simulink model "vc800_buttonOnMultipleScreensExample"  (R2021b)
settings: Solver=FixedStepDiscrete  StartTime=0.0  StopTime=10.0  FixedStep=0.01  RelTol=1e-3  EnableMultiTasking=on
PreLoadFcn:
  | try, model_open; catch, disp('Error occurred while executing model pre-load callback: model_open.m'); disp('Please assure that the MATLAB working directory is set to the model directory before opening.'); end
InitFcn:
  | try, model_open; catch, end
model workspace (MAT data in the model file):
  IOScreen_Label_XCoord = 1
  IOScreen_Row1_YCoord = 1
  IOScreen_Row2_YCoord = 12
  IOScreen_Value_XCoord = 110
  MainScreen_Row1_YCoord = 7
  MainScreen_Row2_YCoord = 23
  MainScreen_Symbols_XCoord = 1
  MainScreen_Units_XCoord = 69
  MainScreen_Value_XCoord = 64
undefined symbols (not defined in the file or in its folder): case, curr_screen, default, DISP, filtering, gesture, hex2dec, Mode, No, raptor_get_buildNum, raptor_get_safe_string, raptor_hwexp, raptor_xcp_function, Screens, VC800, Voltage
libraries: Raptor_display_lib x190, Raptor_lib x97, simulink_extras x11, Raptor_Datalogging_lib x10, simulink x2
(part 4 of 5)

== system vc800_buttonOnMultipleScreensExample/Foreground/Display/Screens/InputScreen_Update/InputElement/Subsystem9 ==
  y_start_offset : Inport
  x : Inport  Port=2
  In3 : Inport  Port=3
  in_value : Inport  Port=4
  Add22 : Sum
  Constant26 : Constant  Value=40  OutDataTypeStr=int32
  display_draw_text13 : Raptor_display_lib/Drawing Functions/display_draw_text  textPort=off  textVal=in_nam  colorPort=off  col=FFFF  opacity=100  font=Future  fontFile=''  heightPort=off  height=20  hAlign=Right  vAlign=Center  spacing=0  layer=Background  pnPort=off
  display_draw_text14 : Raptor_display_lib/Drawing Functions/display_draw_text  textPort=on  textVal='Input1'  colorPort=off  col=FFFF  opacity=100  font=Future  fontFile=''  heightPort=off  height=20  hAlign=Left  vAlign=Center  spacing=0  layer=Background  pnPort=off
  raptor_string : Raptor_lib/Strings/raptor_string  stringName=''  string=''  dynamicSize=Fixed Size  strSize=10  storage=Volatile (RAM)  calVisible=off  calAccess=4  strFunction=raptor_xcp_function(gcb)
  raptor_string_printf : Raptor_lib/Strings/raptor_string_printf  formatString='%u'
  y_end_offset : Outport  VectorParamsAs1DForOutWhenUnconnected=off
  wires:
  raptor_string/1 -> raptor_string_printf/1
  Add22/1 -> display_draw_text13/2, y_end_offset/1, display_draw_text14/2
  In3/1 -> display_draw_text14/1
  raptor_string_printf/1 -> display_draw_text14/3
  y_start_offset/1 -> Add22/1
  Constant26/1 -> Add22/2
  in_value/1 -> raptor_string_printf/2
  x/1 -> display_draw_text13/1

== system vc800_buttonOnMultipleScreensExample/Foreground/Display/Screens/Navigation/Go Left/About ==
  Action Port : ActionPort  ActionPortLabel=case [ 5 ]:
  display_goto_screen : Raptor_display_lib/Screen Functions/display_goto_screen  screenPort=off  ScreenName='MainScreen'

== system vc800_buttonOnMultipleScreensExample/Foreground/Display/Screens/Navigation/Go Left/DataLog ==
  Action Port : ActionPort  ActionPortLabel=case [ 4 ]:
  display_goto_screen : Raptor_display_lib/Screen Functions/display_goto_screen  screenPort=off  ScreenName='AboutScreen'

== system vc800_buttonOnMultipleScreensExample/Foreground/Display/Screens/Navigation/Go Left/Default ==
  Action Port : ActionPort  ActionPortLabel=default:
  display_goto_screen : Raptor_display_lib/Screen Functions/display_goto_screen  screenPort=off  ScreenName='MainScreen'

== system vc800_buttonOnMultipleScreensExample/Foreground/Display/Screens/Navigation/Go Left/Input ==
  Action Port : ActionPort  ActionPortLabel=case [ 2 ]:
  display_goto_screen : Raptor_display_lib/Screen Functions/display_goto_screen  screenPort=off  ScreenName='OutputScreen'

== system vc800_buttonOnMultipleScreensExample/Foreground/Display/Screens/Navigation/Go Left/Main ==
  Action Port : ActionPort  ActionPortLabel=case [ 1 ]:
  display_goto_screen : Raptor_display_lib/Screen Functions/display_goto_screen  screenPort=off  ScreenName='InputScreen'

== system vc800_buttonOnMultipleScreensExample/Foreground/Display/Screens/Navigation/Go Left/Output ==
  Action Port : ActionPort  ActionPortLabel=case [ 3 ]:
  display_goto_screen : Raptor_display_lib/Screen Functions/display_goto_screen  screenPort=off  ScreenName='DataLogScreen'

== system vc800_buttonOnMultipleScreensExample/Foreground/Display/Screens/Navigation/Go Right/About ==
  Action Port : ActionPort  ActionPortLabel=case [ 5 ]:
  display_goto_screen : Raptor_display_lib/Screen Functions/display_goto_screen  screenPort=off  ScreenName='DataLogScreen'

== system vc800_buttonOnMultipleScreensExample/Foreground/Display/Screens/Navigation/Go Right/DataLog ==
  Action Port : ActionPort  ActionPortLabel=case [ 4 ]:
  display_goto_screen : Raptor_display_lib/Screen Functions/display_goto_screen  screenPort=off  ScreenName='OutputScreen'

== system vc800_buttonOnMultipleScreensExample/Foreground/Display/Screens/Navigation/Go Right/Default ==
  Action Port : ActionPort  ActionPortLabel=default:
  display_goto_screen : Raptor_display_lib/Screen Functions/display_goto_screen  screenPort=off  ScreenName='MainScreen'

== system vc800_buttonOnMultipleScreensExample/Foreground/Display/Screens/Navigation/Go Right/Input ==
  Action Port : ActionPort  ActionPortLabel=case [ 2 ]:
  display_goto_screen : Raptor_display_lib/Screen Functions/display_goto_screen  screenPort=off  ScreenName='MainScreen'

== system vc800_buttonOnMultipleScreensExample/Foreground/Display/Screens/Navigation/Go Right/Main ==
  Action Port : ActionPort  ActionPortLabel=case [ 1 ]:
  display_goto_screen : Raptor_display_lib/Screen Functions/display_goto_screen  screenPort=off  ScreenName='AboutScreen'

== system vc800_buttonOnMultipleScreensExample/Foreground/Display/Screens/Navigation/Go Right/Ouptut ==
  Action Port : ActionPort  ActionPortLabel=case [ 3 ]:
  display_goto_screen : Raptor_display_lib/Screen Functions/display_goto_screen  screenPort=off  ScreenName='InputScreen'

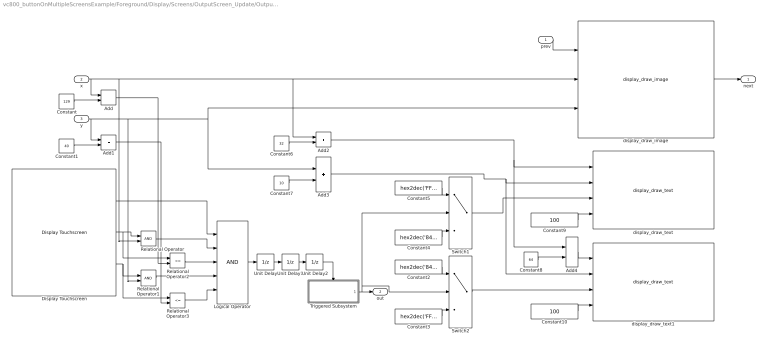
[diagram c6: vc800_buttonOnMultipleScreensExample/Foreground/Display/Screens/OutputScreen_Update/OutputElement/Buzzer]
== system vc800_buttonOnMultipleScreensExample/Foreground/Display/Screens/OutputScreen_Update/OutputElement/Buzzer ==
  prev : Inport
  x : Inport  Port=2
  y : Inport  Port=3
  Add{,1..4} (5 alike) : Sum
  Constant : Constant  Value=129
  Constant1 : Constant  Value=40
  Constant10 : Constant  Value=100  OutDataTypeStr=uint32
  Constant2 : Constant  Value=hex2dec('8410')  OutDataTypeStr=uint16
  Constant3 : Constant  Value=hex2dec('FFFF')  OutDataTypeStr=uint16
  Constant4 : Constant  Value=hex2dec('8410')  OutDataTypeStr=uint16
  Constant5 : Constant  Value=hex2dec('FFFF')  OutDataTypeStr=uint16
  Constant6 : Constant  Value=32  OutDataTypeStr=int32
  Constant7 : Constant  Value=10  OutDataTypeStr=int32
  Constant8 : Constant  Value=64  OutDataTypeStr=int32
  Constant9 : Constant  Value=100  OutDataTypeStr=uint32
  Display Touchscreen : Raptor_display_lib/Touchscreen/Display Touchscreen
  Logical Operator : Logic  Inputs=5  IconShape=distinctive  AllPortsSameDT=off  OutDataTypeStr=boolean
  Relational Operator : RelationalOperator  OutDataTypeStr=boolean
  Relational Operator1 : RelationalOperator  OutDataTypeStr=boolean
  Relational Operator2 : RelationalOperator  Operator=<=  OutDataTypeStr=boolean
  Relational Operator3 : RelationalOperator  Operator=<=  OutDataTypeStr=boolean
  Switch1 : Switch  Criteria=u2 ~= 0
  Switch2 : Switch  Criteria=u2 ~= 0
  Triggered Subsystem : Subsystem  TreatAsAtomicUnit=on
  Unit Delay : UnitDelay  SampleTime=-1  HasFrameUpgradeWarning=on
  Unit Delay1 : UnitDelay  InitialCondition=1  SampleTime=-1  HasFrameUpgradeWarning=on
  Unit Delay2 : UnitDelay  SampleTime=-1  HasFrameUpgradeWarning=on
  display_draw_image : Raptor_display_lib/Drawing Functions/display_draw_image  imagePort=off  imageFile=toggle_frame.png  opacityPort=off  opacity=100  drawMode=Draw Entire Image  alpha=Draw as Transparent  layer=Background  drawModeXY=Top Left  pnPort=on
  display_draw_text : Raptor_display_lib/Drawing Functions/display_draw_text  textPort=off  textVal='On'  colorPort=on  col=8410  opacity=100  font=Future  fontFile=''  heightPort=off  height=20  hAlign=Center  vAlign=Top  spacing=0  layer=Background  pnPort=off
  display_draw_text1 : Raptor_display_lib/Drawing Functions/display_draw_text  textPort=off  textVal='Off'  colorPort=on  col=FFFF  opacity=100  font=Future  fontFile=''  heightPort=off  height=20  hAlign=Center  vAlign=Top  spacing=0  layer=Background  pnPort=off
  next : Outport  VectorParamsAs1DForOutWhenUnconnected=off
  out : Outport  Port=2  VectorParamsAs1DForOutWhenUnconnected=off
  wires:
  x/1 -> Add/1, Relational Operator/2, Add2/1, display_draw_image/2
  Display Touchscreen/2 -> Relational Operator/1, Relational Operator2/1
  Display Touchscreen/3 -> Relational Operator1/1, Relational Operator3/1
  y/1 -> Add1/1, Relational Operator1/2, Add3/1, display_draw_image/3
  Constant/1 -> Add/2
  Constant1/1 -> Add1/2
  Add/1 -> Relational Operator2/2
  Add1/1 -> Relational Operator3/2
  Relational Operator3/1 -> Logical Operator/5
  Relational Operator1/1 -> Logical Operator/4
  Relational Operator2/1 -> Logical Operator/3
  Relational Operator/1 -> Logical Operator/2
  Display Touchscreen/1 -> Logical Operator/1
  Unit Delay1/1 -> Unit Delay2/1
  Unit Delay/1 -> Unit Delay1/1
  Logical Operator/1 -> Unit Delay/1
  Unit Delay2/1 -> Triggered Subsystem/Trigger
  prev/1 -> display_draw_image/1
  display_draw_image/1 -> next/1
  Triggered Subsystem/1(Out1) -> Switch1/2, Switch2/2, out/1
  Switch1/1 -> display_draw_text/3
  Switch2/1 -> display_draw_text1/3
  Constant2/1 -> Switch2/1
  Constant4/1 -> Switch1/3
  Constant3/1 -> Switch2/3
  Constant5/1 -> Switch1/1
  Constant6/1 -> Add2/2
  Add2/1 -> Add4/1, display_draw_text/1
  Constant7/1 -> Add3/2
  Add3/1 -> display_draw_text/2, display_draw_text1/2
  Constant8/1 -> Add4/2
  Add4/1 -> display_draw_text1/1
  Constant9/1 -> display_draw_text/4
  Constant10/1 -> display_draw_text1/4

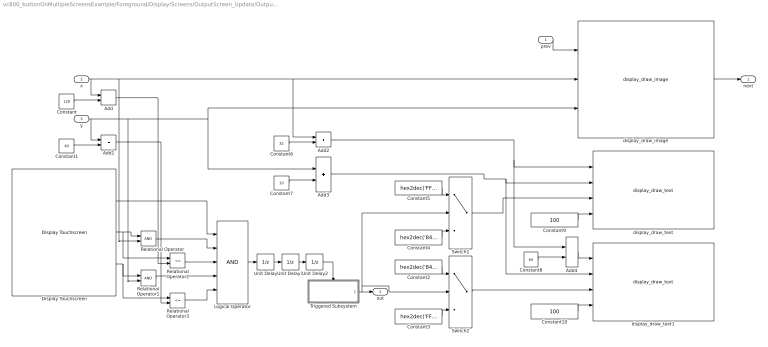
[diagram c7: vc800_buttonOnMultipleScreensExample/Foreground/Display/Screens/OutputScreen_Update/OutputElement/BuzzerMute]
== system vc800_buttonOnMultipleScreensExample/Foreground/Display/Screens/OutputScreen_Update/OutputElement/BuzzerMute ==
  prev : Inport
  x : Inport  Port=2
  y : Inport  Port=3
  Add{,1..4} (5 alike) : Sum
  Constant : Constant  Value=129
  Constant1 : Constant  Value=40
  Constant10 : Constant  Value=100  OutDataTypeStr=uint32
  Constant2 : Constant  Value=hex2dec('8410')  OutDataTypeStr=uint16
  Constant3 : Constant  Value=hex2dec('FFFF')  OutDataTypeStr=uint16
  Constant4 : Constant  Value=hex2dec('8410')  OutDataTypeStr=uint16
  Constant5 : Constant  Value=hex2dec('FFFF')  OutDataTypeStr=uint16
  Constant6 : Constant  Value=32  OutDataTypeStr=int32
  Constant7 : Constant  Value=10  OutDataTypeStr=int32
  Constant8 : Constant  Value=64  OutDataTypeStr=int32
  Constant9 : Constant  Value=100  OutDataTypeStr=uint32
  Display Touchscreen : Raptor_display_lib/Touchscreen/Display Touchscreen
  Logical Operator : Logic  Inputs=5  IconShape=distinctive  AllPortsSameDT=off  OutDataTypeStr=boolean
  Relational Operator : RelationalOperator  OutDataTypeStr=boolean
  Relational Operator1 : RelationalOperator  OutDataTypeStr=boolean
  Relational Operator2 : RelationalOperator  Operator=<=  OutDataTypeStr=boolean
  Relational Operator3 : RelationalOperator  Operator=<=  OutDataTypeStr=boolean
  Switch1 : Switch  Criteria=u2 ~= 0
  Switch2 : Switch  Criteria=u2 ~= 0
  Triggered Subsystem : Subsystem  TreatAsAtomicUnit=on
  Unit Delay : UnitDelay  SampleTime=-1  HasFrameUpgradeWarning=on
  Unit Delay1 : UnitDelay  InitialCondition=1  SampleTime=-1  HasFrameUpgradeWarning=on
  Unit Delay2 : UnitDelay  SampleTime=-1  HasFrameUpgradeWarning=on
  display_draw_image : Raptor_display_lib/Drawing Functions/display_draw_image  imagePort=off  imageFile=toggle_frame.png  opacityPort=off  opacity=100  drawMode=Draw Entire Image  alpha=Draw as Transparent  layer=Background  drawModeXY=Top Left  pnPort=on
  display_draw_text : Raptor_display_lib/Drawing Functions/display_draw_text  textPort=off  textVal='On'  colorPort=on  col=8410  opacity=100  font=Future  fontFile=''  heightPort=off  height=20  hAlign=Center  vAlign=Top  spacing=0  layer=Background  pnPort=off
  display_draw_text1 : Raptor_display_lib/Drawing Functions/display_draw_text  textPort=off  textVal='Off'  colorPort=on  col=FFFF  opacity=100  font=Future  fontFile=''  heightPort=off  height=20  hAlign=Center  vAlign=Top  spacing=0  layer=Background  pnPort=off
  next : Outport  VectorParamsAs1DForOutWhenUnconnected=off
  out : Outport  Port=2  VectorParamsAs1DForOutWhenUnconnected=off
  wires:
  Constant10/1 -> display_draw_text1/4
  Constant9/1 -> display_draw_text/4
  Add4/1 -> display_draw_text1/1
  Constant8/1 -> Add4/2
  Add3/1 -> display_draw_text1/2, display_draw_text/2
  Constant7/1 -> Add3/2
  Add2/1 -> display_draw_text/1, Add4/1
  Constant6/1 -> Add2/2
  Constant5/1 -> Switch1/1
  Constant3/1 -> Switch2/3
  Constant4/1 -> Switch1/3
  Constant2/1 -> Switch2/1
  Switch2/1 -> display_draw_text1/3
  Switch1/1 -> display_draw_text/3
  Triggered Subsystem/1(Out1) -> out/1, Switch2/2, Switch1/2
  display_draw_image/1 -> next/1
  prev/1 -> display_draw_image/1
  Unit Delay2/1 -> Triggered Subsystem/Trigger
  Logical Operator/1 -> Unit Delay/1
  Unit Delay/1 -> Unit Delay1/1
  Unit Delay1/1 -> Unit Delay2/1
  Display Touchscreen/1 -> Logical Operator/1
  Relational Operator/1 -> Logical Operator/2
  Relational Operator2/1 -> Logical Operator/3
  Relational Operator1/1 -> Logical Operator/4
  Relational Operator3/1 -> Logical Operator/5
  Add1/1 -> Relational Operator3/2
  Add/1 -> Relational Operator2/2
  Constant1/1 -> Add1/2
  Constant/1 -> Add/2
  y/1 -> display_draw_image/3, Add3/1, Relational Operator1/2, Add1/1
  Display Touchscreen/3 -> Relational Operator3/1, Relational Operator1/1
  Display Touchscreen/2 -> Relational Operator2/1, Relational Operator/1
  x/1 -> display_draw_image/2, Add2/1, Relational Operator/2, Add/1

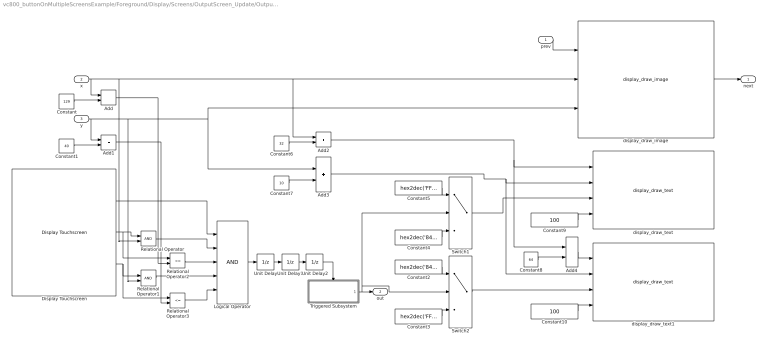
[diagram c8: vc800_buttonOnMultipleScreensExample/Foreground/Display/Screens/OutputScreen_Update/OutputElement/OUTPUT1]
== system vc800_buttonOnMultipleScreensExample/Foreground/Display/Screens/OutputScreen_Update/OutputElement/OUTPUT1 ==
  prev : Inport
  x : Inport  Port=2
  y : Inport  Port=3
  Add{,1..4} (5 alike) : Sum
  Constant : Constant  Value=129
  Constant1 : Constant  Value=40
  Constant10 : Constant  Value=100  OutDataTypeStr=uint32
  Constant2 : Constant  Value=hex2dec('8410')  OutDataTypeStr=uint16
  Constant3 : Constant  Value=hex2dec('FFFF')  OutDataTypeStr=uint16
  Constant4 : Constant  Value=hex2dec('8410')  OutDataTypeStr=uint16
  Constant5 : Constant  Value=hex2dec('FFFF')  OutDataTypeStr=uint16
  Constant6 : Constant  Value=32  OutDataTypeStr=int32
  Constant7 : Constant  Value=10  OutDataTypeStr=int32
  Constant8 : Constant  Value=64  OutDataTypeStr=int32
  Constant9 : Constant  Value=100  OutDataTypeStr=uint32
  Display Touchscreen : Raptor_display_lib/Touchscreen/Display Touchscreen
  Logical Operator : Logic  Inputs=5  IconShape=distinctive  AllPortsSameDT=off  OutDataTypeStr=boolean
  Relational Operator : RelationalOperator  OutDataTypeStr=boolean
  Relational Operator1 : RelationalOperator  OutDataTypeStr=boolean
  Relational Operator2 : RelationalOperator  Operator=<=  OutDataTypeStr=boolean
  Relational Operator3 : RelationalOperator  Operator=<=  OutDataTypeStr=boolean
  Switch1 : Switch  Criteria=u2 ~= 0
  Switch2 : Switch  Criteria=u2 ~= 0
  Triggered Subsystem : Subsystem  TreatAsAtomicUnit=on
  Unit Delay : UnitDelay  SampleTime=-1  HasFrameUpgradeWarning=on
  Unit Delay1 : UnitDelay  InitialCondition=1  SampleTime=-1  HasFrameUpgradeWarning=on
  Unit Delay2 : UnitDelay  SampleTime=-1  HasFrameUpgradeWarning=on
  display_draw_image : Raptor_display_lib/Drawing Functions/display_draw_image  imagePort=off  imageFile=toggle_frame.png  opacityPort=off  opacity=100  drawMode=Draw Entire Image  alpha=Draw as Transparent  layer=Background  drawModeXY=Top Left  pnPort=on
  display_draw_text : Raptor_display_lib/Drawing Functions/display_draw_text  textPort=off  textVal='On'  colorPort=on  col=8410  opacity=100  font=Future  fontFile=''  heightPort=off  height=20  hAlign=Center  vAlign=Top  spacing=0  layer=Background  pnPort=off
  display_draw_text1 : Raptor_display_lib/Drawing Functions/display_draw_text  textPort=off  textVal='Off'  colorPort=on  col=FFFF  opacity=100  font=Future  fontFile=''  heightPort=off  height=20  hAlign=Center  vAlign=Top  spacing=0  layer=Background  pnPort=off
  next : Outport  VectorParamsAs1DForOutWhenUnconnected=off
  out : Outport  Port=2  VectorParamsAs1DForOutWhenUnconnected=off
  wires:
  x/1 -> Add/1, Relational Operator/2, Add2/1, display_draw_image/2
  Display Touchscreen/2 -> Relational Operator/1, Relational Operator2/1
  Display Touchscreen/3 -> Relational Operator1/1, Relational Operator3/1
  y/1 -> Add1/1, Relational Operator1/2, Add3/1, display_draw_image/3
  Constant/1 -> Add/2
  Constant1/1 -> Add1/2
  Add/1 -> Relational Operator2/2
  Add1/1 -> Relational Operator3/2
  Relational Operator3/1 -> Logical Operator/5
  Relational Operator1/1 -> Logical Operator/4
  Relational Operator2/1 -> Logical Operator/3
  Relational Operator/1 -> Logical Operator/2
  Display Touchscreen/1 -> Logical Operator/1
  Unit Delay1/1 -> Unit Delay2/1
  Unit Delay/1 -> Unit Delay1/1
  Logical Operator/1 -> Unit Delay/1
  Unit Delay2/1 -> Triggered Subsystem/Trigger
  prev/1 -> display_draw_image/1
  display_draw_image/1 -> next/1
  Triggered Subsystem/1(Out1) -> Switch1/2, Switch2/2, out/1
  Switch1/1 -> display_draw_text/3
  Switch2/1 -> display_draw_text1/3
  Constant2/1 -> Switch2/1
  Constant4/1 -> Switch1/3
  Constant3/1 -> Switch2/3
  Constant5/1 -> Switch1/1
  Constant6/1 -> Add2/2
  Add2/1 -> Add4/1, display_draw_text/1
  Constant7/1 -> Add3/2
  Add3/1 -> display_draw_text/2, display_draw_text1/2
  Constant8/1 -> Add4/2
  Add4/1 -> display_draw_text1/1
  Constant9/1 -> display_draw_text/4
  Constant10/1 -> display_draw_text1/4

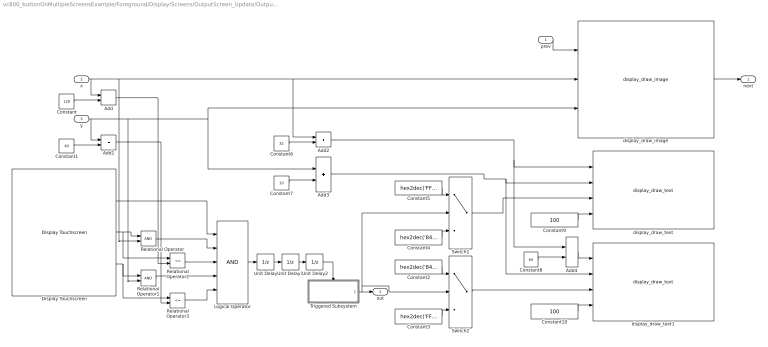
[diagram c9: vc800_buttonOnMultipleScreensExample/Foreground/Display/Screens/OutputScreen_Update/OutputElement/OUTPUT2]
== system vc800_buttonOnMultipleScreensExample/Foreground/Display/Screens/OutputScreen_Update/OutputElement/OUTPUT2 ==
  prev : Inport
  x : Inport  Port=2
  y : Inport  Port=3
  Add{,1..4} (5 alike) : Sum
  Constant : Constant  Value=129
  Constant1 : Constant  Value=40
  Constant10 : Constant  Value=100  OutDataTypeStr=uint32
  Constant2 : Constant  Value=hex2dec('8410')  OutDataTypeStr=uint16
  Constant3 : Constant  Value=hex2dec('FFFF')  OutDataTypeStr=uint16
  Constant4 : Constant  Value=hex2dec('8410')  OutDataTypeStr=uint16
  Constant5 : Constant  Value=hex2dec('FFFF')  OutDataTypeStr=uint16
  Constant6 : Constant  Value=32  OutDataTypeStr=int32
  Constant7 : Constant  Value=10  OutDataTypeStr=int32
  Constant8 : Constant  Value=64  OutDataTypeStr=int32
  Constant9 : Constant  Value=100  OutDataTypeStr=uint32
  Display Touchscreen : Raptor_display_lib/Touchscreen/Display Touchscreen
  Logical Operator : Logic  Inputs=5  IconShape=distinctive  AllPortsSameDT=off  OutDataTypeStr=boolean
  Relational Operator : RelationalOperator  OutDataTypeStr=boolean
  Relational Operator1 : RelationalOperator  OutDataTypeStr=boolean
  Relational Operator2 : RelationalOperator  Operator=<=  OutDataTypeStr=boolean
  Relational Operator3 : RelationalOperator  Operator=<=  OutDataTypeStr=boolean
  Switch1 : Switch  Criteria=u2 ~= 0
  Switch2 : Switch  Criteria=u2 ~= 0
  Triggered Subsystem : Subsystem  TreatAsAtomicUnit=on
  Unit Delay : UnitDelay  SampleTime=-1  HasFrameUpgradeWarning=on
  Unit Delay1 : UnitDelay  InitialCondition=1  SampleTime=-1  HasFrameUpgradeWarning=on
  Unit Delay2 : UnitDelay  SampleTime=-1  HasFrameUpgradeWarning=on
  display_draw_image : Raptor_display_lib/Drawing Functions/display_draw_image  imagePort=off  imageFile=toggle_frame.png  opacityPort=off  opacity=100  drawMode=Draw Entire Image  alpha=Draw as Transparent  layer=Background  drawModeXY=Top Left  pnPort=on
  display_draw_text : Raptor_display_lib/Drawing Functions/display_draw_text  textPort=off  textVal='On'  colorPort=on  col=8410  opacity=100  font=Future  fontFile=''  heightPort=off  height=20  hAlign=Center  vAlign=Top  spacing=0  layer=Background  pnPort=off
  display_draw_text1 : Raptor_display_lib/Drawing Functions/display_draw_text  textPort=off  textVal='Off'  colorPort=on  col=FFFF  opacity=100  font=Future  fontFile=''  heightPort=off  height=20  hAlign=Center  vAlign=Top  spacing=0  layer=Background  pnPort=off
  next : Outport  VectorParamsAs1DForOutWhenUnconnected=off
  out : Outport  Port=2  VectorParamsAs1DForOutWhenUnconnected=off
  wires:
  Constant10/1 -> display_draw_text1/4
  Constant9/1 -> display_draw_text/4
  Add4/1 -> display_draw_text1/1
  Constant8/1 -> Add4/2
  Add3/1 -> display_draw_text1/2, display_draw_text/2
  Constant7/1 -> Add3/2
  Add2/1 -> display_draw_text/1, Add4/1
  Constant6/1 -> Add2/2
  Constant5/1 -> Switch1/1
  Constant3/1 -> Switch2/3
  Constant4/1 -> Switch1/3
  Constant2/1 -> Switch2/1
  Switch2/1 -> display_draw_text1/3
  Switch1/1 -> display_draw_text/3
  Triggered Subsystem/1(Out1) -> out/1, Switch2/2, Switch1/2
  display_draw_image/1 -> next/1
  prev/1 -> display_draw_image/1
  Unit Delay2/1 -> Triggered Subsystem/Trigger
  Logical Operator/1 -> Unit Delay/1
  Unit Delay/1 -> Unit Delay1/1
  Unit Delay1/1 -> Unit Delay2/1
  Display Touchscreen/1 -> Logical Operator/1
  Relational Operator/1 -> Logical Operator/2
  Relational Operator2/1 -> Logical Operator/3
  Relational Operator1/1 -> Logical Operator/4
  Relational Operator3/1 -> Logical Operator/5
  Add1/1 -> Relational Operator3/2
  Add/1 -> Relational Operator2/2
  Constant1/1 -> Add1/2
  Constant/1 -> Add/2
  y/1 -> display_draw_image/3, Add3/1, Relational Operator1/2, Add1/1
  Display Touchscreen/3 -> Relational Operator3/1, Relational Operator1/1
  Display Touchscreen/2 -> Relational Operator2/1, Relational Operator/1
  x/1 -> display_draw_image/2, Add2/1, Relational Operator/2, Add/1

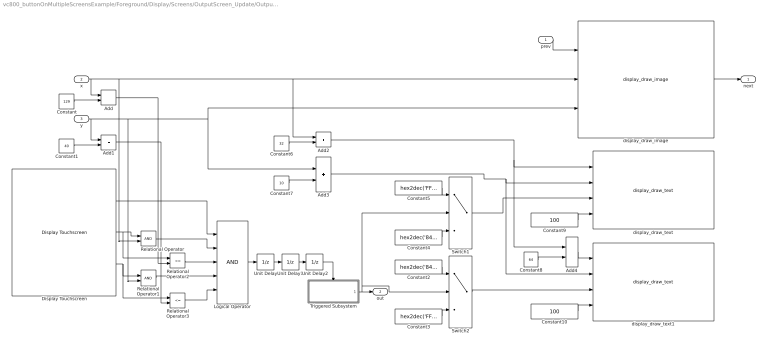
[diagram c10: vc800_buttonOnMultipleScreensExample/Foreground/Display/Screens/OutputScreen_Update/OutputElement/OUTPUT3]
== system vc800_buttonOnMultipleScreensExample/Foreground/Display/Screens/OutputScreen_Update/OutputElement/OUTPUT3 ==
  prev : Inport
  x : Inport  Port=2
  y : Inport  Port=3
  Add{,1..4} (5 alike) : Sum
  Constant : Constant  Value=129
  Constant1 : Constant  Value=40
  Constant10 : Constant  Value=100  OutDataTypeStr=uint32
  Constant2 : Constant  Value=hex2dec('8410')  OutDataTypeStr=uint16
  Constant3 : Constant  Value=hex2dec('FFFF')  OutDataTypeStr=uint16
  Constant4 : Constant  Value=hex2dec('8410')  OutDataTypeStr=uint16
  Constant5 : Constant  Value=hex2dec('FFFF')  OutDataTypeStr=uint16
  Constant6 : Constant  Value=32  OutDataTypeStr=int32
  Constant7 : Constant  Value=10  OutDataTypeStr=int32
  Constant8 : Constant  Value=64  OutDataTypeStr=int32
  Constant9 : Constant  Value=100  OutDataTypeStr=uint32
  Display Touchscreen : Raptor_display_lib/Touchscreen/Display Touchscreen
  Logical Operator : Logic  Inputs=5  IconShape=distinctive  AllPortsSameDT=off  OutDataTypeStr=boolean
  Relational Operator : RelationalOperator  OutDataTypeStr=boolean
  Relational Operator1 : RelationalOperator  OutDataTypeStr=boolean
  Relational Operator2 : RelationalOperator  Operator=<=  OutDataTypeStr=boolean
  Relational Operator3 : RelationalOperator  Operator=<=  OutDataTypeStr=boolean
  Switch1 : Switch  Criteria=u2 ~= 0
  Switch2 : Switch  Criteria=u2 ~= 0
  Triggered Subsystem : Subsystem  TreatAsAtomicUnit=on
  Unit Delay : UnitDelay  SampleTime=-1  HasFrameUpgradeWarning=on
  Unit Delay1 : UnitDelay  InitialCondition=1  SampleTime=-1  HasFrameUpgradeWarning=on
  Unit Delay2 : UnitDelay  SampleTime=-1  HasFrameUpgradeWarning=on
  display_draw_image : Raptor_display_lib/Drawing Functions/display_draw_image  imagePort=off  imageFile=toggle_frame.png  opacityPort=off  opacity=100  drawMode=Draw Entire Image  alpha=Draw as Transparent  layer=Background  drawModeXY=Top Left  pnPort=on
  display_draw_text : Raptor_display_lib/Drawing Functions/display_draw_text  textPort=off  textVal='On'  colorPort=on  col=8410  opacity=100  font=Future  fontFile=''  heightPort=off  height=20  hAlign=Center  vAlign=Top  spacing=0  layer=Background  pnPort=off
  display_draw_text1 : Raptor_display_lib/Drawing Functions/display_draw_text  textPort=off  textVal='Off'  colorPort=on  col=FFFF  opacity=100  font=Future  fontFile=''  heightPort=off  height=20  hAlign=Center  vAlign=Top  spacing=0  layer=Background  pnPort=off
  next : Outport  VectorParamsAs1DForOutWhenUnconnected=off
  out : Outport  Port=2  VectorParamsAs1DForOutWhenUnconnected=off
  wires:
  x/1 -> Add/1, Relational Operator/2, Add2/1, display_draw_image/2
  Display Touchscreen/2 -> Relational Operator/1, Relational Operator2/1
  Display Touchscreen/3 -> Relational Operator1/1, Relational Operator3/1
  y/1 -> Add1/1, Relational Operator1/2, Add3/1, display_draw_image/3
  Constant/1 -> Add/2
  Constant1/1 -> Add1/2
  Add/1 -> Relational Operator2/2
  Add1/1 -> Relational Operator3/2
  Relational Operator3/1 -> Logical Operator/5
  Relational Operator1/1 -> Logical Operator/4
  Relational Operator2/1 -> Logical Operator/3
  Relational Operator/1 -> Logical Operator/2
  Display Touchscreen/1 -> Logical Operator/1
  Unit Delay1/1 -> Unit Delay2/1
  Unit Delay/1 -> Unit Delay1/1
  Logical Operator/1 -> Unit Delay/1
  Unit Delay2/1 -> Triggered Subsystem/Trigger
  prev/1 -> display_draw_image/1
  display_draw_image/1 -> next/1
  Triggered Subsystem/1(Out1) -> Switch1/2, Switch2/2, out/1
  Switch1/1 -> display_draw_text/3
  Switch2/1 -> display_draw_text1/3
  Constant2/1 -> Switch2/1
  Constant4/1 -> Switch1/3
  Constant3/1 -> Switch2/3
  Constant5/1 -> Switch1/1
  Constant6/1 -> Add2/2
  Add2/1 -> Add4/1, display_draw_text/1
  Constant7/1 -> Add3/2
  Add3/1 -> display_draw_text/2, display_draw_text1/2
  Constant8/1 -> Add4/2
  Add4/1 -> display_draw_text1/1
  Constant9/1 -> display_draw_text/4
  Constant10/1 -> display_draw_text1/4

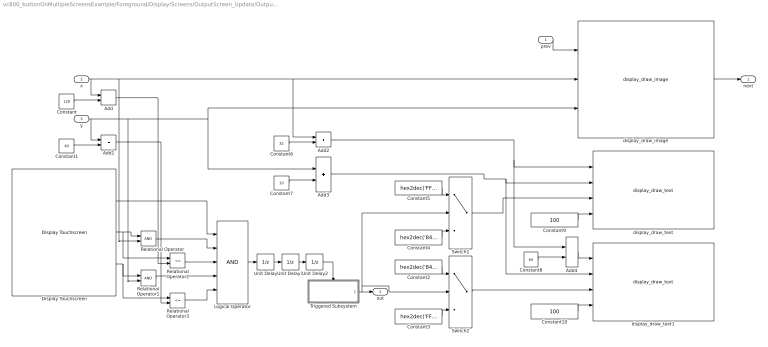
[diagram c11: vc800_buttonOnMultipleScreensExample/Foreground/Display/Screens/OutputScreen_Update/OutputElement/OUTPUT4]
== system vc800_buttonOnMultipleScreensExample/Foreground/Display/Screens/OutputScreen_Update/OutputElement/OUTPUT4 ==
  prev : Inport
  x : Inport  Port=2
  y : Inport  Port=3
  Add{,1..4} (5 alike) : Sum
  Constant : Constant  Value=129
  Constant1 : Constant  Value=40
  Constant10 : Constant  Value=100  OutDataTypeStr=uint32
  Constant2 : Constant  Value=hex2dec('8410')  OutDataTypeStr=uint16
  Constant3 : Constant  Value=hex2dec('FFFF')  OutDataTypeStr=uint16
  Constant4 : Constant  Value=hex2dec('8410')  OutDataTypeStr=uint16
  Constant5 : Constant  Value=hex2dec('FFFF')  OutDataTypeStr=uint16
  Constant6 : Constant  Value=32  OutDataTypeStr=int32
  Constant7 : Constant  Value=10  OutDataTypeStr=int32
  Constant8 : Constant  Value=64  OutDataTypeStr=int32
  Constant9 : Constant  Value=100  OutDataTypeStr=uint32
  Display Touchscreen : Raptor_display_lib/Touchscreen/Display Touchscreen
  Logical Operator : Logic  Inputs=5  IconShape=distinctive  AllPortsSameDT=off  OutDataTypeStr=boolean
  Relational Operator : RelationalOperator  OutDataTypeStr=boolean
  Relational Operator1 : RelationalOperator  OutDataTypeStr=boolean
  Relational Operator2 : RelationalOperator  Operator=<=  OutDataTypeStr=boolean
  Relational Operator3 : RelationalOperator  Operator=<=  OutDataTypeStr=boolean
  Switch1 : Switch  Criteria=u2 ~= 0
  Switch2 : Switch  Criteria=u2 ~= 0
  Triggered Subsystem : Subsystem  TreatAsAtomicUnit=on
  Unit Delay : UnitDelay  SampleTime=-1  HasFrameUpgradeWarning=on
  Unit Delay1 : UnitDelay  InitialCondition=1  SampleTime=-1  HasFrameUpgradeWarning=on
  Unit Delay2 : UnitDelay  SampleTime=-1  HasFrameUpgradeWarning=on
  display_draw_image : Raptor_display_lib/Drawing Functions/display_draw_image  imagePort=off  imageFile=toggle_frame.png  opacityPort=off  opacity=100  drawMode=Draw Entire Image  alpha=Draw as Transparent  layer=Background  drawModeXY=Top Left  pnPort=on
  display_draw_text : Raptor_display_lib/Drawing Functions/display_draw_text  textPort=off  textVal='On'  colorPort=on  col=8410  opacity=100  font=Future  fontFile=''  heightPort=off  height=20  hAlign=Center  vAlign=Top  spacing=0  layer=Background  pnPort=off
  display_draw_text1 : Raptor_display_lib/Drawing Functions/display_draw_text  textPort=off  textVal='Off'  colorPort=on  col=FFFF  opacity=100  font=Future  fontFile=''  heightPort=off  height=20  hAlign=Center  vAlign=Top  spacing=0  layer=Background  pnPort=off
  next : Outport  VectorParamsAs1DForOutWhenUnconnected=off
  out : Outport  Port=2  VectorParamsAs1DForOutWhenUnconnected=off
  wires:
  Constant10/1 -> display_draw_text1/4
  Constant9/1 -> display_draw_text/4
  Add4/1 -> display_draw_text1/1
  Constant8/1 -> Add4/2
  Add3/1 -> display_draw_text1/2, display_draw_text/2
  Constant7/1 -> Add3/2
  Add2/1 -> display_draw_text/1, Add4/1
  Constant6/1 -> Add2/2
  Constant5/1 -> Switch1/1
  Constant3/1 -> Switch2/3
  Constant4/1 -> Switch1/3
  Constant2/1 -> Switch2/1
  Switch2/1 -> display_draw_text1/3
  Switch1/1 -> display_draw_text/3
  Triggered Subsystem/1(Out1) -> out/1, Switch2/2, Switch1/2
  display_draw_image/1 -> next/1
  prev/1 -> display_draw_image/1
  Unit Delay2/1 -> Triggered Subsystem/Trigger
  Logical Operator/1 -> Unit Delay/1
  Unit Delay/1 -> Unit Delay1/1
  Unit Delay1/1 -> Unit Delay2/1
  Display Touchscreen/1 -> Logical Operator/1
  Relational Operator/1 -> Logical Operator/2
  Relational Operator2/1 -> Logical Operator/3
  Relational Operator1/1 -> Logical Operator/4
  Relational Operator3/1 -> Logical Operator/5
  Add1/1 -> Relational Operator3/2
  Add/1 -> Relational Operator2/2
  Constant1/1 -> Add1/2
  Constant/1 -> Add/2
  y/1 -> display_draw_image/3, Add3/1, Relational Operator1/2, Add1/1
  Display Touchscreen/3 -> Relational Operator3/1, Relational Operator1/1
  Display Touchscreen/2 -> Relational Operator2/1, Relational Operator/1
  x/1 -> display_draw_image/2, Add2/1, Relational Operator/2, Add/1

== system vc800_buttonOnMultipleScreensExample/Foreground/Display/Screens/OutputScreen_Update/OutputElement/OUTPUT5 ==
  prev : Inport
  x : Inport  Port=2
  y : Inport  Port=3
  Add{,1..4} (5 alike) : Sum
  Constant : Constant  Value=129
  Constant1 : Constant  Value=40
  Constant10 : Constant  Value=100  OutDataTypeStr=uint32
  Constant2 : Constant  Value=hex2dec('8410')  OutDataTypeStr=uint16
  Constant3 : Constant  Value=hex2dec('FFFF')  OutDataTypeStr=uint16
  Constant4 : Constant  Value=hex2dec('8410')  OutDataTypeStr=uint16
  Constant5 : Constant  Value=hex2dec('FFFF')  OutDataTypeStr=uint16
  Constant6 : Constant  Value=32  OutDataTypeStr=int32
  Constant7 : Constant  Value=10  OutDataTypeStr=int32
  Constant8 : Constant  Value=64  OutDataTypeStr=int32
  Constant9 : Constant  Value=100  OutDataTypeStr=uint32
  Display Touchscreen : Raptor_display_lib/Touchscreen/Display Touchscreen
  Logical Operator : Logic  Inputs=5  IconShape=distinctive  AllPortsSameDT=off  OutDataTypeStr=boolean
  Relational Operator : RelationalOperator  OutDataTypeStr=boolean
  Relational Operator1 : RelationalOperator  OutDataTypeStr=boolean
  Relational Operator2 : RelationalOperator  Operator=<=  OutDataTypeStr=boolean
  Relational Operator3 : RelationalOperator  Operator=<=  OutDataTypeStr=boolean
  Switch1 : Switch  Criteria=u2 ~= 0
  Switch2 : Switch  Criteria=u2 ~= 0
  Triggered Subsystem : Subsystem  TreatAsAtomicUnit=on
  Unit Delay : UnitDelay  SampleTime=-1  HasFrameUpgradeWarning=on
  Unit Delay1 : UnitDelay  InitialCondition=1  SampleTime=-1  HasFrameUpgradeWarning=on
  Unit Delay2 : UnitDelay  SampleTime=-1  HasFrameUpgradeWarning=on
  display_draw_image : Raptor_display_lib/Drawing Functions/display_draw_image  imagePort=off  imageFile=toggle_frame.png  opacityPort=off  opacity=100  drawMode=Draw Entire Image  alpha=Draw as Transparent  layer=Background  drawModeXY=Top Left  pnPort=on
  display_draw_text : Raptor_display_lib/Drawing Functions/display_draw_text  textPort=off  textVal='On'  colorPort=on  col=8410  opacity=100  font=Future  fontFile=''  heightPort=off  height=20  hAlign=Center  vAlign=Top  spacing=0  layer=Background  pnPort=off
  display_draw_text1 : Raptor_display_lib/Drawing Functions/display_draw_text  textPort=off  textVal='Off'  colorPort=on  col=FFFF  opacity=100  font=Future  fontFile=''  heightPort=off  height=20  hAlign=Center  vAlign=Top  spacing=0  layer=Background  pnPort=off
  next : Outport  VectorParamsAs1DForOutWhenUnconnected=off
  out : Outport  Port=2  VectorParamsAs1DForOutWhenUnconnected=off
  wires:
  x/1 -> Add/1, Relational Operator/2, Add2/1, display_draw_image/2
  Display Touchscreen/2 -> Relational Operator/1, Relational Operator2/1
  Display Touchscreen/3 -> Relational Operator1/1, Relational Operator3/1
  y/1 -> Add1/1, Relational Operator1/2, Add3/1, display_draw_image/3
  Constant/1 -> Add/2
  Constant1/1 -> Add1/2
  Add/1 -> Relational Operator2/2
  Add1/1 -> Relational Operator3/2
  Relational Operator3/1 -> Logical Operator/5
  Relational Operator1/1 -> Logical Operator/4
  Relational Operator2/1 -> Logical Operator/3
  Relational Operator/1 -> Logical Operator/2
  Display Touchscreen/1 -> Logical Operator/1
  Unit Delay1/1 -> Unit Delay2/1
  Unit Delay/1 -> Unit Delay1/1
  Logical Operator/1 -> Unit Delay/1
  Unit Delay2/1 -> Triggered Subsystem/Trigger
  prev/1 -> display_draw_image/1
  display_draw_image/1 -> next/1
  Triggered Subsystem/1(Out1) -> Switch1/2, Switch2/2, out/1
  Switch1/1 -> display_draw_text/3
  Switch2/1 -> display_draw_text1/3
  Constant2/1 -> Switch2/1
  Constant4/1 -> Switch1/3
  Constant3/1 -> Switch2/3
  Constant5/1 -> Switch1/1
  Constant6/1 -> Add2/2
  Add2/1 -> Add4/1, display_draw_text/1
  Constant7/1 -> Add3/2
  Add3/1 -> display_draw_text/2, display_draw_text1/2
  Constant8/1 -> Add4/2
  Add4/1 -> display_draw_text1/1
  Constant9/1 -> display_draw_text/4
  Constant10/1 -> display_draw_text1/4

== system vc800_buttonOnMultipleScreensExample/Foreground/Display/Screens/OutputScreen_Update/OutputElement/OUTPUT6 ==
  prev : Inport
  x : Inport  Port=2
  y : Inport  Port=3
  Add{,1..4} (5 alike) : Sum
  Constant : Constant  Value=129
  Constant1 : Constant  Value=40
  Constant10 : Constant  Value=100  OutDataTypeStr=uint32
  Constant2 : Constant  Value=hex2dec('8410')  OutDataTypeStr=uint16
  Constant3 : Constant  Value=hex2dec('FFFF')  OutDataTypeStr=uint16
  Constant4 : Constant  Value=hex2dec('8410')  OutDataTypeStr=uint16
  Constant5 : Constant  Value=hex2dec('FFFF')  OutDataTypeStr=uint16
  Constant6 : Constant  Value=32  OutDataTypeStr=int32
  Constant7 : Constant  Value=10  OutDataTypeStr=int32
  Constant8 : Constant  Value=64  OutDataTypeStr=int32
  Constant9 : Constant  Value=100  OutDataTypeStr=uint32
  Display Touchscreen : Raptor_display_lib/Touchscreen/Display Touchscreen
  Logical Operator : Logic  Inputs=5  IconShape=distinctive  AllPortsSameDT=off  OutDataTypeStr=boolean
  Relational Operator : RelationalOperator  OutDataTypeStr=boolean
  Relational Operator1 : RelationalOperator  OutDataTypeStr=boolean
  Relational Operator2 : RelationalOperator  Operator=<=  OutDataTypeStr=boolean
  Relational Operator3 : RelationalOperator  Operator=<=  OutDataTypeStr=boolean
  Switch1 : Switch  Criteria=u2 ~= 0
  Switch2 : Switch  Criteria=u2 ~= 0
  Triggered Subsystem : Subsystem  TreatAsAtomicUnit=on
  Unit Delay : UnitDelay  SampleTime=-1  HasFrameUpgradeWarning=on
  Unit Delay1 : UnitDelay  InitialCondition=1  SampleTime=-1  HasFrameUpgradeWarning=on
  Unit Delay2 : UnitDelay  SampleTime=-1  HasFrameUpgradeWarning=on
  display_draw_image : Raptor_display_lib/Drawing Functions/display_draw_image  imagePort=off  imageFile=toggle_frame.png  opacityPort=off  opacity=100  drawMode=Draw Entire Image  alpha=Draw as Transparent  layer=Background  drawModeXY=Top Left  pnPort=on
  display_draw_text : Raptor_display_lib/Drawing Functions/display_draw_text  textPort=off  textVal='On'  colorPort=on  col=8410  opacity=100  font=Future  fontFile=''  heightPort=off  height=20  hAlign=Center  vAlign=Top  spacing=0  layer=Background  pnPort=off
  display_draw_text1 : Raptor_display_lib/Drawing Functions/display_draw_text  textPort=off  textVal='Off'  colorPort=on  col=FFFF  opacity=100  font=Future  fontFile=''  heightPort=off  height=20  hAlign=Center  vAlign=Top  spacing=0  layer=Background  pnPort=off
  next : Outport  VectorParamsAs1DForOutWhenUnconnected=off
  out : Outport  Port=2  VectorParamsAs1DForOutWhenUnconnected=off
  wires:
  Constant10/1 -> display_draw_text1/4
  Constant9/1 -> display_draw_text/4
  Add4/1 -> display_draw_text1/1
  Constant8/1 -> Add4/2
  Add3/1 -> display_draw_text1/2, display_draw_text/2
  Constant7/1 -> Add3/2
  Add2/1 -> display_draw_text/1, Add4/1
  Constant6/1 -> Add2/2
  Constant5/1 -> Switch1/1
  Constant3/1 -> Switch2/3
  Constant4/1 -> Switch1/3
  Constant2/1 -> Switch2/1
  Switch2/1 -> display_draw_text1/3
  Switch1/1 -> display_draw_text/3
  Triggered Subsystem/1(Out1) -> out/1, Switch2/2, Switch1/2
  display_draw_image/1 -> next/1
  prev/1 -> display_draw_image/1
  Unit Delay2/1 -> Triggered Subsystem/Trigger
  Logical Operator/1 -> Unit Delay/1
  Unit Delay/1 -> Unit Delay1/1
  Unit Delay1/1 -> Unit Delay2/1
  Display Touchscreen/1 -> Logical Operator/1
  Relational Operator/1 -> Logical Operator/2
  Relational Operator2/1 -> Logical Operator/3
  Relational Operator1/1 -> Logical Operator/4
  Relational Operator3/1 -> Logical Operator/5
  Add1/1 -> Relational Operator3/2
  Add/1 -> Relational Operator2/2
  Constant1/1 -> Add1/2
  Constant/1 -> Add/2
  y/1 -> display_draw_image/3, Add3/1, Relational Operator1/2, Add1/1
  Display Touchscreen/3 -> Relational Operator3/1, Relational Operator1/1
  Display Touchscreen/2 -> Relational Operator2/1, Relational Operator/1
  x/1 -> display_draw_image/2, Add2/1, Relational Operator/2, Add/1

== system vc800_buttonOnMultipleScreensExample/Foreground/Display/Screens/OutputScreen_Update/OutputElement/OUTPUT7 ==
  prev : Inport
  x : Inport  Port=2
  y : Inport  Port=3
  Add{,1..4} (5 alike) : Sum
  Constant : Constant  Value=129
  Constant1 : Constant  Value=40
  Constant10 : Constant  Value=100  OutDataTypeStr=uint32
  Constant2 : Constant  Value=hex2dec('8410')  OutDataTypeStr=uint16
  Constant3 : Constant  Value=hex2dec('FFFF')  OutDataTypeStr=uint16
  Constant4 : Constant  Value=hex2dec('8410')  OutDataTypeStr=uint16
  Constant5 : Constant  Value=hex2dec('FFFF')  OutDataTypeStr=uint16
  Constant6 : Constant  Value=32  OutDataTypeStr=int32
  Constant7 : Constant  Value=10  OutDataTypeStr=int32
  Constant8 : Constant  Value=64  OutDataTypeStr=int32
  Constant9 : Constant  Value=100  OutDataTypeStr=uint32
  Display Touchscreen : Raptor_display_lib/Touchscreen/Display Touchscreen
  Logical Operator : Logic  Inputs=5  IconShape=distinctive  AllPortsSameDT=off  OutDataTypeStr=boolean
  Relational Operator : RelationalOperator  OutDataTypeStr=boolean
  Relational Operator1 : RelationalOperator  OutDataTypeStr=boolean
  Relational Operator2 : RelationalOperator  Operator=<=  OutDataTypeStr=boolean
  Relational Operator3 : RelationalOperator  Operator=<=  OutDataTypeStr=boolean
  Switch1 : Switch  Criteria=u2 ~= 0
  Switch2 : Switch  Criteria=u2 ~= 0
  Triggered Subsystem : Subsystem  TreatAsAtomicUnit=on
  Unit Delay : UnitDelay  SampleTime=-1  HasFrameUpgradeWarning=on
  Unit Delay1 : UnitDelay  InitialCondition=1  SampleTime=-1  HasFrameUpgradeWarning=on
  Unit Delay2 : UnitDelay  SampleTime=-1  HasFrameUpgradeWarning=on
  display_draw_image : Raptor_display_lib/Drawing Functions/display_draw_image  imagePort=off  imageFile=toggle_frame.png  opacityPort=off  opacity=100  drawMode=Draw Entire Image  alpha=Draw as Transparent  layer=Background  drawModeXY=Top Left  pnPort=on
  display_draw_text : Raptor_display_lib/Drawing Functions/display_draw_text  textPort=off  textVal='On'  colorPort=on  col=8410  opacity=100  font=Future  fontFile=''  heightPort=off  height=20  hAlign=Center  vAlign=Top  spacing=0  layer=Background  pnPort=off
  display_draw_text1 : Raptor_display_lib/Drawing Functions/display_draw_text  textPort=off  textVal='Off'  colorPort=on  col=FFFF  opacity=100  font=Future  fontFile=''  heightPort=off  height=20  hAlign=Center  vAlign=Top  spacing=0  layer=Background  pnPort=off
  next : Outport  VectorParamsAs1DForOutWhenUnconnected=off
  out : Outport  Port=2  VectorParamsAs1DForOutWhenUnconnected=off
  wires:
  x/1 -> Add/1, Relational Operator/2, Add2/1, display_draw_image/2
  Display Touchscreen/2 -> Relational Operator/1, Relational Operator2/1
  Display Touchscreen/3 -> Relational Operator1/1, Relational Operator3/1
  y/1 -> Add1/1, Relational Operator1/2, Add3/1, display_draw_image/3
  Constant/1 -> Add/2
  Constant1/1 -> Add1/2
  Add/1 -> Relational Operator2/2
  Add1/1 -> Relational Operator3/2
  Relational Operator3/1 -> Logical Operator/5
  Relational Operator1/1 -> Logical Operator/4
  Relational Operator2/1 -> Logical Operator/3
  Relational Operator/1 -> Logical Operator/2
  Display Touchscreen/1 -> Logical Operator/1
  Unit Delay1/1 -> Unit Delay2/1
  Unit Delay/1 -> Unit Delay1/1
  Logical Operator/1 -> Unit Delay/1
  Unit Delay2/1 -> Triggered Subsystem/Trigger
  prev/1 -> display_draw_image/1
  display_draw_image/1 -> next/1
  Triggered Subsystem/1(Out1) -> Switch1/2, Switch2/2, out/1
  Switch1/1 -> display_draw_text/3
  Switch2/1 -> display_draw_text1/3
  Constant2/1 -> Switch2/1
  Constant4/1 -> Switch1/3
  Constant3/1 -> Switch2/3
  Constant5/1 -> Switch1/1
  Constant6/1 -> Add2/2
  Add2/1 -> Add4/1, display_draw_text/1
  Constant7/1 -> Add3/2
  Add3/1 -> display_draw_text/2, display_draw_text1/2
  Constant8/1 -> Add4/2
  Add4/1 -> display_draw_text1/1
  Constant9/1 -> display_draw_text/4
  Constant10/1 -> display_draw_text1/4

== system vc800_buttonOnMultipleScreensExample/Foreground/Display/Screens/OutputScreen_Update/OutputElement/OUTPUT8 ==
  prev : Inport
  x : Inport  Port=2
  y : Inport  Port=3
  Add{,1..4} (5 alike) : Sum
  Constant : Constant  Value=129
  Constant1 : Constant  Value=40
  Constant10 : Constant  Value=100  OutDataTypeStr=uint32
  Constant2 : Constant  Value=hex2dec('8410')  OutDataTypeStr=uint16
  Constant3 : Constant  Value=hex2dec('FFFF')  OutDataTypeStr=uint16
  Constant4 : Constant  Value=hex2dec('8410')  OutDataTypeStr=uint16
  Constant5 : Constant  Value=hex2dec('FFFF')  OutDataTypeStr=uint16
  Constant6 : Constant  Value=32  OutDataTypeStr=int32
  Constant7 : Constant  Value=10  OutDataTypeStr=int32
  Constant8 : Constant  Value=64  OutDataTypeStr=int32
  Constant9 : Constant  Value=100  OutDataTypeStr=uint32
  Display Touchscreen : Raptor_display_lib/Touchscreen/Display Touchscreen
  Logical Operator : Logic  Inputs=5  IconShape=distinctive  AllPortsSameDT=off  OutDataTypeStr=boolean
  Relational Operator : RelationalOperator  OutDataTypeStr=boolean
  Relational Operator1 : RelationalOperator  OutDataTypeStr=boolean
  Relational Operator2 : RelationalOperator  Operator=<=  OutDataTypeStr=boolean
  Relational Operator3 : RelationalOperator  Operator=<=  OutDataTypeStr=boolean
  Switch1 : Switch  Criteria=u2 ~= 0
  Switch2 : Switch  Criteria=u2 ~= 0
  Triggered Subsystem : Subsystem  TreatAsAtomicUnit=on
  Unit Delay : UnitDelay  SampleTime=-1  HasFrameUpgradeWarning=on
  Unit Delay1 : UnitDelay  InitialCondition=1  SampleTime=-1  HasFrameUpgradeWarning=on
  Unit Delay2 : UnitDelay  SampleTime=-1  HasFrameUpgradeWarning=on
  display_draw_image : Raptor_display_lib/Drawing Functions/display_draw_image  imagePort=off  imageFile=toggle_frame.png  opacityPort=off  opacity=100  drawMode=Draw Entire Image  alpha=Draw as Transparent  layer=Background  drawModeXY=Top Left  pnPort=on
  display_draw_text : Raptor_display_lib/Drawing Functions/display_draw_text  textPort=off  textVal='On'  colorPort=on  col=8410  opacity=100  font=Future  fontFile=''  heightPort=off  height=20  hAlign=Center  vAlign=Top  spacing=0  layer=Background  pnPort=off
  display_draw_text1 : Raptor_display_lib/Drawing Functions/display_draw_text  textPort=off  textVal='Off'  colorPort=on  col=FFFF  opacity=100  font=Future  fontFile=''  heightPort=off  height=20  hAlign=Center  vAlign=Top  spacing=0  layer=Background  pnPort=off
  next : Outport  VectorParamsAs1DForOutWhenUnconnected=off
  out : Outport  Port=2  VectorParamsAs1DForOutWhenUnconnected=off
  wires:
  Constant10/1 -> display_draw_text1/4
  Constant9/1 -> display_draw_text/4
  Add4/1 -> display_draw_text1/1
  Constant8/1 -> Add4/2
  Add3/1 -> display_draw_text1/2, display_draw_text/2
  Constant7/1 -> Add3/2
  Add2/1 -> display_draw_text/1, Add4/1
  Constant6/1 -> Add2/2
  Constant5/1 -> Switch1/1
  Constant3/1 -> Switch2/3
  Constant4/1 -> Switch1/3
  Constant2/1 -> Switch2/1
  Switch2/1 -> display_draw_text1/3
  Switch1/1 -> display_draw_text/3
  Triggered Subsystem/1(Out1) -> out/1, Switch2/2, Switch1/2
  display_draw_image/1 -> next/1
  prev/1 -> display_draw_image/1
  Unit Delay2/1 -> Triggered Subsystem/Trigger
  Logical Operator/1 -> Unit Delay/1
  Unit Delay/1 -> Unit Delay1/1
  Unit Delay1/1 -> Unit Delay2/1
  Display Touchscreen/1 -> Logical Operator/1
  Relational Operator/1 -> Logical Operator/2
  Relational Operator2/1 -> Logical Operator/3
  Relational Operator1/1 -> Logical Operator/4
  Relational Operator3/1 -> Logical Operator/5
  Add1/1 -> Relational Operator3/2
  Add/1 -> Relational Operator2/2
  Constant1/1 -> Add1/2
  Constant/1 -> Add/2
  y/1 -> display_draw_image/3, Add3/1, Relational Operator1/2, Add1/1
  Display Touchscreen/3 -> Relational Operator3/1, Relational Operator1/1
  Display Touchscreen/2 -> Relational Operator2/1, Relational Operator/1
  x/1 -> display_draw_image/2, Add2/1, Relational Operator/2, Add/1

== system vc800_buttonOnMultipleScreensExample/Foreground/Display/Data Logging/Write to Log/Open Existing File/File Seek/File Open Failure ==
  file_in : Inport
  Enable : EnablePort
  Constant : Constant  Value=false  OutDataTypeStr=Inherit: Inherit via back propagation
  file_out : Outport  VectorParamsAs1DForOutWhenUnconnected=off
  Success : Outport  Port=2  VectorParamsAs1DForOutWhenUnconnected=off
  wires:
  Constant/1 -> Success/1
  file_in/1 -> file_out/1

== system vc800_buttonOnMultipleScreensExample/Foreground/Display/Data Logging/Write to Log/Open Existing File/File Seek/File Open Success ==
  file_in : Inport
  Enable : EnablePort
  Constant : Constant  Value=0  OutDataTypeStr=Inherit: Inherit via back propagation
  raptor_fileIO_seek1 : Raptor_Datalogging_lib/raptor_fileIO_seek  resourceValues=USB|(None)  resource=USB  seekTypeValues=File Start|Current Location|File End  seekType=3
  file_out : Outport  VectorParamsAs1DForOutWhenUnconnected=off
  Out2 : Outport  Port=2  VectorParamsAs1DForOutWhenUnconnected=off
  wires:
  raptor_fileIO_seek1/1 -> file_out/1
  raptor_fileIO_seek1/2 -> Out2/1
  file_in/1 -> raptor_fileIO_seek1/1
  Constant/1 -> raptor_fileIO_seek1/2

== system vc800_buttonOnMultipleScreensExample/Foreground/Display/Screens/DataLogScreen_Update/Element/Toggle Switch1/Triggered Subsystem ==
  Trigger : TriggerPort  VariantControl=Variant
  Constant2 : Constant
  D Latch : simulink_extras/Flip Flops/D Latch
  Unit Delay : UnitDelay  InitialCondition=InitialCondition  SampleTime=-1  HasFrameUpgradeWarning=on
  Out1 : Outport  VectorParamsAs1DForOutWhenUnconnected=off
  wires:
  D Latch/2 -> Unit Delay/1
  Unit Delay/1 -> D Latch/1
  D Latch/1 -> Out1/1
  Constant2/1 -> D Latch/2

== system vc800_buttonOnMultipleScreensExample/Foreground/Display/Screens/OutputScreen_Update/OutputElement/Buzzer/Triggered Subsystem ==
  Trigger : TriggerPort  VariantControl=Variant
  Constant2 : Constant
  D Latch : simulink_extras/Flip Flops/D Latch
  Unit Delay : UnitDelay  InitialCondition=InitialCondition  SampleTime=-1  HasFrameUpgradeWarning=on
  Out1 : Outport  VectorParamsAs1DForOutWhenUnconnected=off
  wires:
  D Latch/2 -> Unit Delay/1
  Unit Delay/1 -> D Latch/1
  D Latch/1 -> Out1/1
  Constant2/1 -> D Latch/2

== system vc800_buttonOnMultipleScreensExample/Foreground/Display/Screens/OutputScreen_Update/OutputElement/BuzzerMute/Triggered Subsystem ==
  Trigger : TriggerPort  VariantControl=Variant
  Constant2 : Constant
  D Latch : simulink_extras/Flip Flops/D Latch
  Unit Delay : UnitDelay  InitialCondition=InitialCondition  SampleTime=-1  HasFrameUpgradeWarning=on
  Out1 : Outport  VectorParamsAs1DForOutWhenUnconnected=off
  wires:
  Constant2/1 -> D Latch/2
  D Latch/1 -> Out1/1
  Unit Delay/1 -> D Latch/1
  D Latch/2 -> Unit Delay/1

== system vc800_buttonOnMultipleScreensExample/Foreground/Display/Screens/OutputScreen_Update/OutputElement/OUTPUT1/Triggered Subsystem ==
  Trigger : TriggerPort  VariantControl=Variant
  Constant2 : Constant
  D Latch : simulink_extras/Flip Flops/D Latch
  Unit Delay : UnitDelay  InitialCondition=InitialCondition  SampleTime=-1  HasFrameUpgradeWarning=on
  Out1 : Outport  VectorParamsAs1DForOutWhenUnconnected=off
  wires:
  D Latch/2 -> Unit Delay/1
  Unit Delay/1 -> D Latch/1
  D Latch/1 -> Out1/1
  Constant2/1 -> D Latch/2
